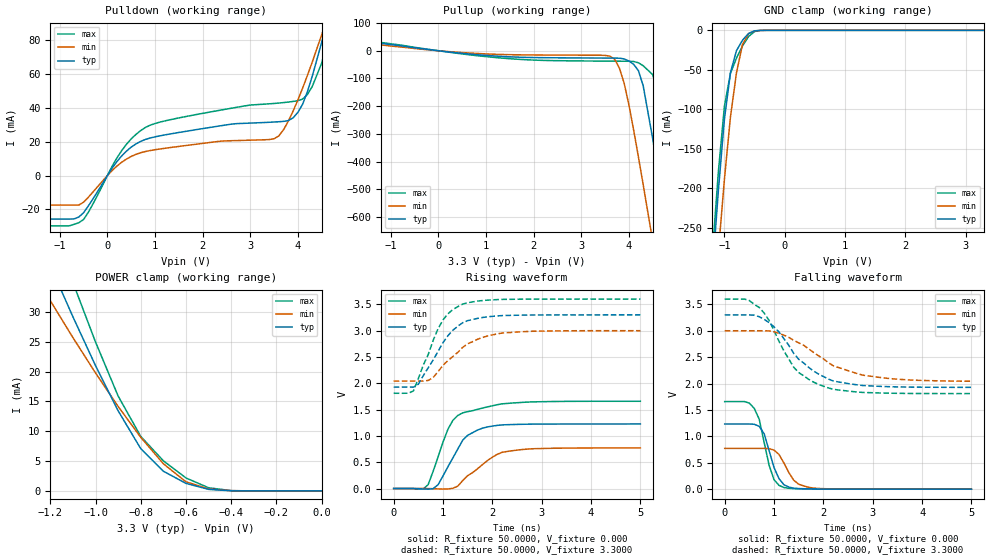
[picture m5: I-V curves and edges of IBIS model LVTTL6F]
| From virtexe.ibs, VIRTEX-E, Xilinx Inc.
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|   Model LVTTL6F
[Model]   LVTTL6F
Model_type   I/O
Polarity   Non-Inverting
Enable   Active-Low
Vinl =   0.800V
Vinh =   2.000V
Vmeas =   1.4000V
Cref =  35.0000pF
Rref =   1.0000M
Vref =  0.000V
C_comp   5.0000pF   4.0000pF   6.0000pF
[Temperature Range]   25.0000   100.0000   0.000
[Voltage Range]   3.3000V   3.0000V   3.6000V
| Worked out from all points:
|   slope of the pulldown table from 0 to 0.495 V, typ, clamps not added: 29.7 ohm
|   slope of the pullup table from 0 to 0.495 V, typ, clamps not added: 53.2 ohm
|   GND clamp passes 1 mA (typ) near -0.51 V on its own axis
|   POWER clamp passes 1 mA (typ) near -0.57 V on its own axis
|   rising waveform, R_fixture 50.0000, V_fixture 0.000: 20-80 % time 464ps typ, 637ps min, 432ps max; typ from 0 V to 1.23 V
|   rising waveform, R_fixture 50.0000, V_fixture 3.3000: 20-80 % time 585ps typ, 727ps min, 502ps max; typ from 1.93 V to 3.3 V
|   falling waveform, R_fixture 50.0000, V_fixture 0.000: 20-80 % time 258ps typ, 293ps min, 245ps max; typ from 1.23 V to 0 V
|   falling waveform, R_fixture 50.0000, V_fixture 3.3000: 20-80 % time 812ps typ, 1.11ns min, 700ps max; typ from 3.3 V to 1.93 V
[Pulldown]
| voltage   I(typ)   I(min)   I(max)
-3.3V     -25.79mA   -17.5mA    -29.79mA
-600mV    -24.57mA   -17.5mA    -27.97mA
-400mV    -18.03mA   -12.85mA   -21.77mA
300mV     11.6mA     7.84mA     14.73mA
800mV     21.38mA    14.22mA    28.48mA
3.5V      31.68mA    21.76mA    42.67mA
3.7V      32.05mA    27.13mA    43.18mA
4V        37.36mA    44.71mA    44.3mA
4.2V      49.6mA     59.21mA    47.98mA
4.5V      78.82mA    83.31mA    66.54mA
4.7V      100.8mA    100.5mA    89.68mA
6.6V      343.9mA    288.4mA    376.2mA
[Pullup]
| voltage   I(typ)   I(min)   I(max)
-3.3V     76.5mA     72.6mA     74.8mA
700mV     -12.61mA   -8.705mA   -15.61mA
3.6V      -26.42mA   -19.41mA   -37.49mA
3.8V      -26.91mA   -62.44mA   -37.69mA
3.9V      -29.44mA   -116.9mA   -37.79mA
4.2V      -71.79mA   -383mA     -43.41mA
4.3V      -126.2mA   -482.7mA   -54.06mA
4.5V      -317.3mA   -687.1mA   -86.33mA
4.7V      -537mA     -895.1mA   -197.6mA
4.9V      -764.2mA   -1.105A    -410.4mA
5.1V      -994.9mA   -1.316A    -641.1mA
6.6V      -2.76A     -2.923A    -2.453A
[GND_clamp]
| voltage   I(typ)   I(min)   I(max)
-3.3V     -2.749A    -2.594A    -2.805A
-1.2V     -306mA     -377.1mA   -282.7mA
-1.1V     -202.5mA   -280mA     -178.8mA
-1V       -112.5mA   -188.5mA   -95.98mA
-900mV    -53.5mA    -109.7mA   -54.53mA
-800mV    -25.67mA   -53.59mA   -35.13mA
-700mV    -12.44mA   -17.88mA   -19.82mA
-600mV    -3.982mA   -4.202mA   -7.865mA
-500mV    -601.5uA   -800.3uA   -1.508mA
-400mV    -51.05uA   -119.3uA   -124.3uA
3.3V      18.74nA    3.634uA    18.92nA
[POWER_clamp]
| voltage   I(typ)   I(min)   I(max)
-3.3V     237mA      175.9mA    284.4mA
-1.3V     46.69mA    38.29mA    56.33mA
-1.2V     37.79mA    31.9mA     45.45mA
-1.1V     29.2mA     25.71mA    34.95mA
-1V       21.01mA    19.78mA    24.97mA
-900mV    13.43mA    14.17mA    15.91mA
-800mV    7.091mA    8.993mA    9.139mA
-700mV    3.305mA    4.554mA    5.052mA
-600mV    1.265mA    1.529mA    2.172mA
-500mV    263.8uA    333.6uA    531.5uA
-400mV    22.63uA    44.12uA    49.77uA
0V        18.8nA     38.3nA     22.53nA
[Ramp]
| variable   typ   min   max
dV/dt_r   0.7362/0.4838n   0.4628/0.6170n   0.9948/0.4203n
dV/dt_f   0.8232/0.8055n   0.5736/1.0818n   1.0740/0.7006n
R_load = 50.0000
[Rising Waveform]
R_fixture = 50.0000
V_fixture = 0.000
| time   V(typ)   V(min)   V(max)
0s        2.953uV    3.405uV    2.844uV
600ps     -9.209mV   241.9uV    -7.69mV
700ps     -12.16mV   -584.3uV   75.02mV
900ps     72.16mV    -7.107mV   599.8mV
1.1ns     414mV      -7.952mV   1.127V
1.2ns     580.7mV    4.816mV    1.294V
1.4ns     918mV      150.6mV    1.438V
1.7ns     1.111V     375.6mV    1.504V
2.2ns     1.208V     688.1mV    1.609V
5ns       1.227V     771.4mV    1.658V
[Rising Waveform]
R_fixture = 50.0000
V_fixture = 3.3000
V_fixture_min = 3.0000
V_fixture_max = 3.6000
| time   V(typ)   V(min)   V(max)
0s        1.927V     2.041V     1.81V
400ps     1.926V     2.042V     1.854V
500ps     1.982V     2.042V     2.088V
700ps     2.293V     2.054V     2.545V
900ps     2.607V     2.22V      3.037V
1ns       2.772V     2.342V     3.204V
1.4ns     3.151V     2.683V     3.505V
1.8ns     3.249V     2.87V      3.572V
2.2ns     3.286V     2.954V     3.594V
5ns       3.3V       2.999V     3.6V
[Falling Waveform]
R_fixture = 50.0000
V_fixture = 0.000
| time   V(typ)   V(min)   V(max)
0s        1.234V     771.5mV    1.658V
400ps     1.234V     771.6mV    1.659V
600ps     1.229V     771.5mV    1.529V
700ps     1.19V      771.7mV    1.325V
800ps     1.049V     772.1mV    883.1mV
1ns       409mV      739.5mV    179.3mV
1.2ns     84.3mV     495.7mV    31.16mV
1.4ns     18.54mV    168.1mV    10mV
1.8ns     5.04mV     21mV       3.7mV
5ns       351.4uV    182uV      309.4uV
[Falling Waveform]
R_fixture = 50.0000
V_fixture = 3.3000
V_fixture_min = 3.0000
V_fixture_max = 3.6000
| time   V(typ)   V(min)   V(max)
0s        3.3V       3V         3.6V
400ps     3.3V       3V         3.6V
700ps     3.267V     3V         3.441V
900ps     3.154V     2.997V     3.195V
1.1ns     2.976V     2.95V      2.801V
1.4ns     2.571V     2.818V     2.308V
1.9ns     2.18V      2.527V     1.984V
2.2ns     2.049V     2.337V     1.891V
2.8ns     1.963V     2.159V     1.832V
5ns       1.928V     2.044V     1.81V
